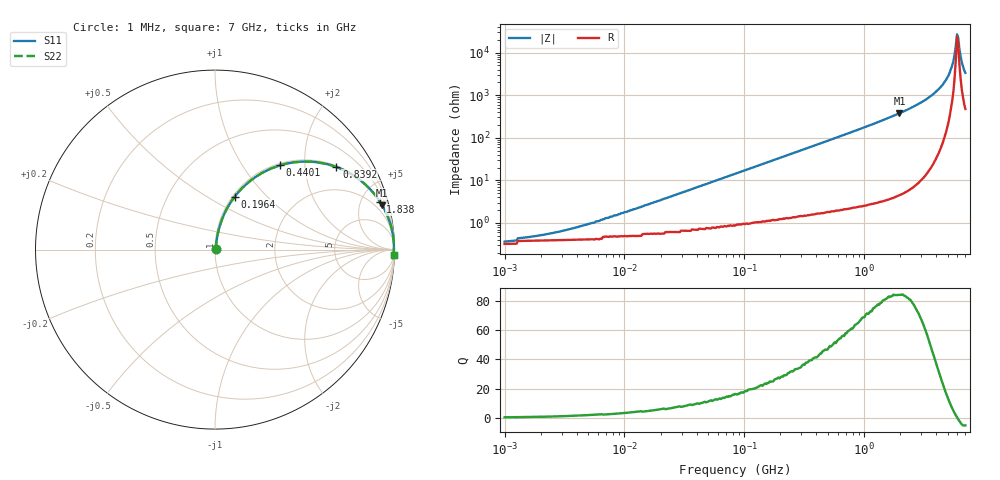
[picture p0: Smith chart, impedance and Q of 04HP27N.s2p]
# MHz S MA R 50
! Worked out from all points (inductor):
!   385 points, 1 MHz to 7 GHz, reference 50 ohm
!   read as one part in series: L = 27 nH near 8.536 MHz
!   highest Q = 83.9 at 1.97 GHz (marker M1), where L = 30.3 nH
!   self-resonance near 5.957 GHz
!   S11 on the Smith chart (normalised r, x): 1 MHz: 1.01, +0.00; 196.4 MHz: 1.02, +0.67; 440.1 MHz: 1.03, +1.50; 839.2 MHz: 1.04, +2.91; 1.838 GHz: 1.09, +6.88; 7 GHz: 11, -65
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1  0.003805 26.3  0.997 -0.1  0.997 -0.1  0.003805 26.3
2.044  0.005057 42.9  0.996 -0.2  0.996 -0.2  0.005057 42.9
4.374  0.008467 60.4  0.996 -0.4  0.996 -0.4  0.008467 60.4
19.575  0.033 78.3  0.994 -1.9  0.994 -1.9  0.033 78.3
85.617  0.143 78.3  0.981 -8.2  0.981 -8.2  0.143 78.3
196.354  0.313 69.7  0.938 -18.2  0.938 -18.2  0.313 69.7
365.931  0.523 57.0  0.839 -31.5  0.839 -31.5  0.523 57.0
440.053  0.594 52.3  0.791 -36.4  0.791 -36.4  0.594 52.3
839.222  0.818 34.3  0.563 -54.8  0.563 -54.8  0.818 34.3
1637.803  0.945 18.4  0.315 -71.0  0.315 -71.0  0.945 18.4
1837.926  0.957 16.2  0.278 -73.2  0.278 -73.2  0.957 16.2
1969.554  0.963 14.9  0.257 -74.4  0.257 -74.4  0.963 14.9
3270.845  0.99 7.2  0.126 -81.8  0.126 -81.8  0.99 7.2
4516.955  0.996 3.2  0.057 -84.3  0.057 -84.3  0.996 3.2
5068.882  0.997 1.9  0.034 -83.5  0.034 -83.5  0.997 1.9
5558.598  0.997 0.9  0.016 -77.9  0.016 -77.9  0.997 0.9
5820.923  0.997 0.4  0.007013 -62.3  0.007013 -62.3  0.997 0.4
5956.691  0.997 0.1  0.003752 -27.2  0.003752 -27.2  0.997 0.1
6095.627  0.997 -0.2  0.004431 38.7  0.004431 38.7  0.997 -0.2
6237.803  0.996 -0.4  0.008113 63.5  0.008113 63.5  0.996 -0.4
6532.181  0.996 -0.9  0.017 75.8  0.017 75.8  0.996 -0.9
7000  0.995 -1.7  0.03 80.1  0.03 80.1  0.995 -1.7
